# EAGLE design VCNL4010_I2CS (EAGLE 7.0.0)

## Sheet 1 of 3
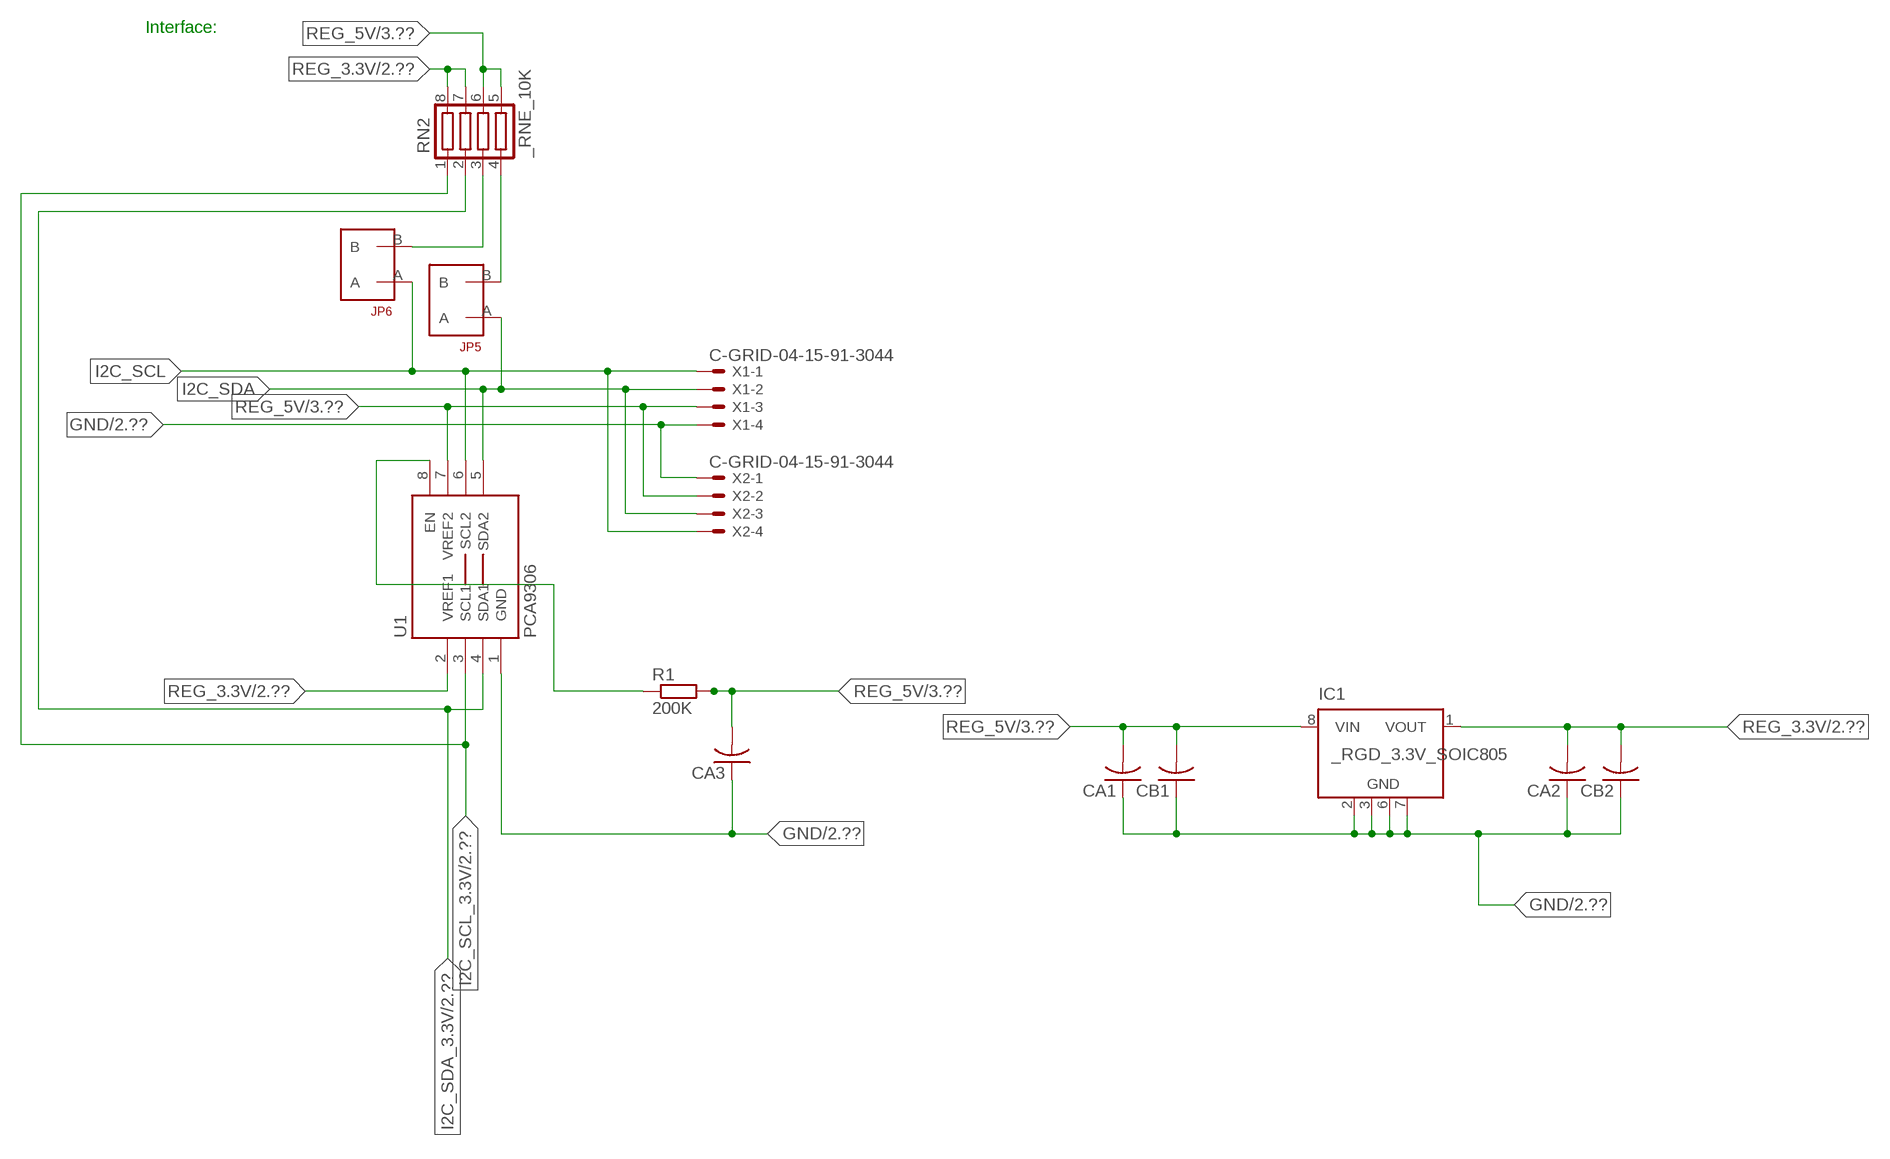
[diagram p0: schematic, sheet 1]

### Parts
CA1  CC1206KRX7R9BB104  [.1UF]
CA2  CC1206KRX7R9BB104  [.1UF]
CA3  CC1206KRX7R9BB104  [.1UF]
CB1  TMK316F106ZL-TC1206K  [TMK316F106ZL-T]
CB2  TMK316F106ZL-TC1206K  [TMK316F106ZL-T]
IC1  _RGD_3.3V_SOIC805  [_RGC_3.3V_SOIC8]
JP5  JUMPER_1X2_2MM  [JUMPER_1X2_2MM]
JP6  JUMPER_1X2_2MM  [JUMPER_1X2_2MM]
R1  200K  RESISTOR_SMT-0603  [R603]
RN2  _RNE_10K  [RNE]
U1  PCA9306  PCA9306_NCD  [PSOP-8]
X1  C-GRID-04-15-91-3044  [15-91-04]
X2  C-GRID-04-15-91-3044  [15-91-04]

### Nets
GND: CA1.1 CA2.1 CA3.1 CB1.1 CB2.1 IC1.2(GND) IC1.3(GND) IC1.6(GND) IC1.7(GND) U1.1(GND) X1.4 X2.1 ; also sheet 2,3
I2C_SCL: JP6.A U1.6(SCL2) X1.1 X2.4
I2C_SCL_3.3V: RN2.1 U1.3(SCL1) ; also sheet 2
I2C_SDA: JP5.A U1.5(SDA2) X1.2 X2.3
I2C_SDA_3.3V: RN2.2 U1.4(SDA1) ; also sheet 2
N$1: JP6.B RN2.3
N$2: JP5.B RN2.4
N$3: R1.1 U1.8(EN)
REG_3.3V: CA2.2 CB2.2 IC1.1(VOUT) RN2.7 RN2.8 U1.2(VREF1) ; also sheet 2
REG_5V: CA1.2 CA3.2 CB1.2 IC1.8(VIN) R1.2 RN2.5 RN2.6 U1.7(VREF2) X1.3 X2.2 ; also sheet 3
Unconnected: IC1.4(NC) IC1.5(NC)

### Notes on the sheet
- Interface:

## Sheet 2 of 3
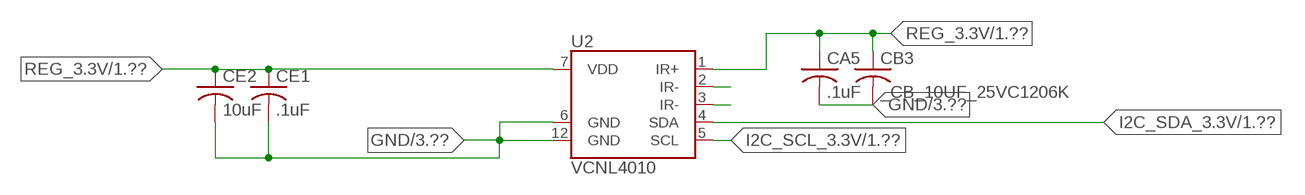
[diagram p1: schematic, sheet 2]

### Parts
CA5  .1uF  CC1206KRX7R9BB104C1206K  [CC1206KRX7R9BB104]
CB3  _CB_10UF_25VC1206K  [_CB_10UF_25V]
CE1  .1uF  _CD_10NF_50VC1206K  [_CD_10NF_50V]
CE2  10uF  CC0603JRNPO8BN1020603  [CC0603JRNPO8BN102]
U2  VCNL4010  VCNL4000  [VCNL4000]

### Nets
GND: CA5.2 CB3.2 CE1.2 CE2.2 U2.6(GND) U2.12(GND) ; also sheet 1,3
I2C_SCL_3.3V: U2.5(SCL) ; also sheet 1
I2C_SDA_3.3V: U2.4(SDA) ; also sheet 1
IR2-: U2.2(IR-)
IR3-: U2.3(IR-)
REG_3.3V: CA5.1 CB3.1 CE1.1 CE2.1 U2.1(IR+) U2.7(VDD) ; also sheet 1

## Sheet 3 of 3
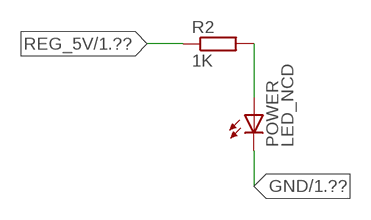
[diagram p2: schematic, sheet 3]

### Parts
POWER  LED_NCD  [CHIPLED_0603]
R2  1K  RESISTOR_SMT-0402  [R402]

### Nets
GND: POWER.C ; also sheet 1,2
N$4: POWER.A R2.2
REG_5V: R2.1 ; also sheet 1

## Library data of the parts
CA1-CA3 CA5 = NCD_ULTIMATE_LIBRARY:CC1206KRX7R9BB104: Capacitor CA .1uF 50V SMT C1206K CC1206KRX7R9BB104
CB1 CB2 = NCD_ULTIMATE_LIBRARY:TMK316F106ZL-T: Capacitor CB 10uF SMT 1206 TMK316F106ZL-T
CB3 = NCD_ULTIMATE_LIBRARY:_CB_10UF_25V: Capacitor 10uF SMT
CE1 = NCD_ULTIMATE_LIBRARY:_CD_10NF_50V: Capacitor 10nF SMT
CE2 = NCD_ULTIMATE_LIBRARY:CC0603JRNPO8BN102: Capacitor CE 1uF SMT CC0603JRNPO8BN102 0603
IC1 = NCD_ULTIMATE_LIBRARY:_RGD_3.3V_SOIC8: Regulator Linear 3.3V Chip Positive VOLTAGE REGULATOR Digikey 497-1199-2-ND/L78L33ACD13TR
JP5 JP6 = NCD_ULTIMATE_CONNECTORS:JUMPER_1X2_2MM
POWER = NCD_ULTIMATE_LIBRARY:LED_NCD: LED Digikey 754-1132-2-ND/APT2012SRCPRV
R1 R2 = NCD_ULTIMATE_LIBRARY:RESISTOR_SMT: NCD Resistor
RN2 = NCD_ULTIMATE_LIBRARY:_RNE_10K: Resistor Array RNE SMT 10K x 4 Single Resistor Source: http://www.ctscorp.com/components/Datasheets/CTSChipArrayDs.pdf Digikey 742C083103JPTR-ND/742C083103JP; OC_FARNELL: unknown; OC_NEWARK: unknown
U1 = NCD_ULTIMATE_LIBRARY:PCA9306_NCD: NCD Bidirectional I2C level shifter. NOT compatible with all available part number pinout schemes- DOUBLE CHECK!!!; PROD_ID: IC-10023
U2 = NCD_ULTIMATE_bhaskar:VCNL4000: Digikey 751-1505-1-ND/VCNL4000-GS08 Fully integrated proximity and ambient light sensor with infrared emitter and I2C interface
X1 X2 = NCD_ULTIMATE_CONNECTORS:C-GRID-04: CONNECTOR 4-Pos I2C wire to board 2.54 mm (0.100") pitch header Digikey WM1342-ND/0015912045; OC_FARNELL: unknown; OC_NEWARK: unknown

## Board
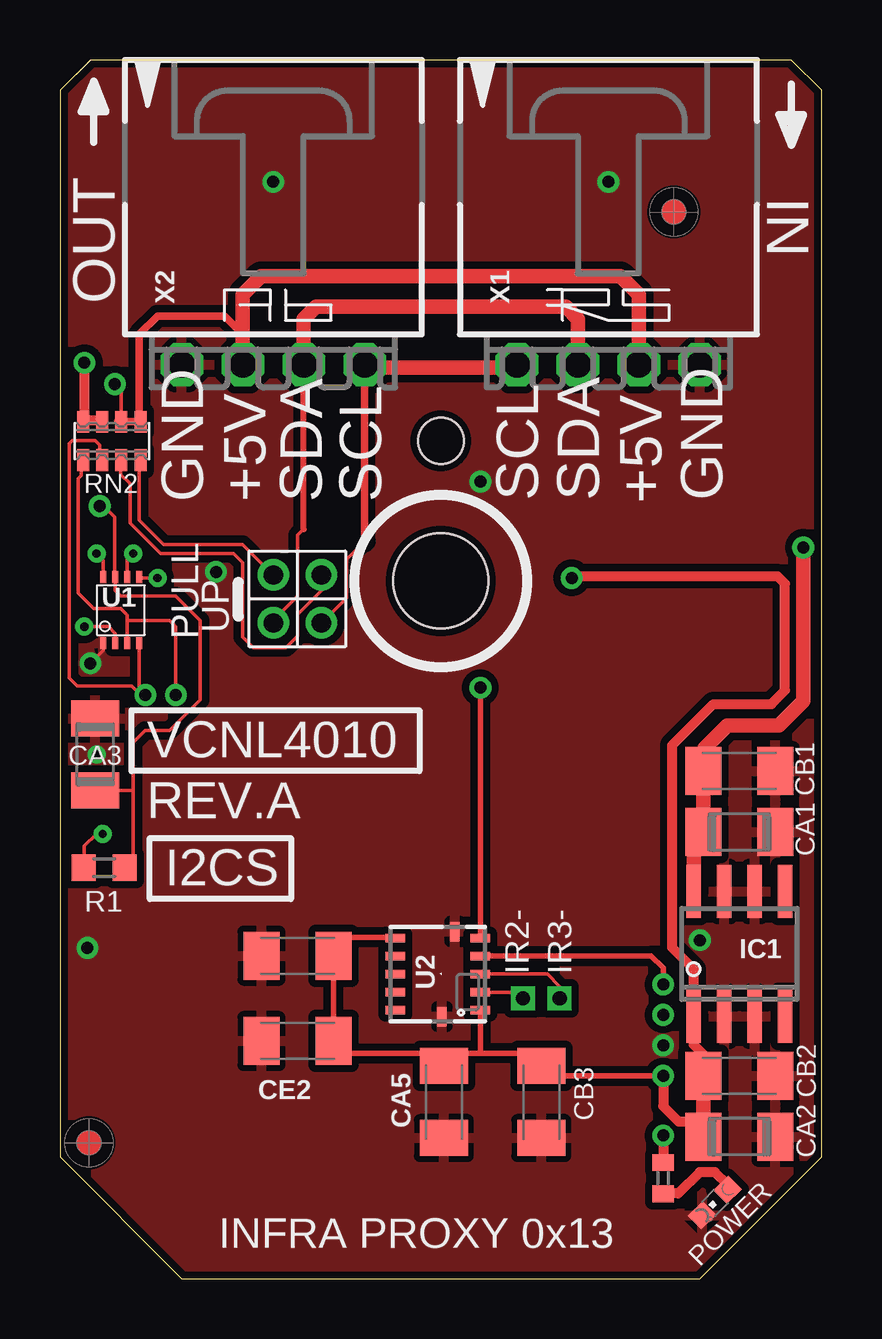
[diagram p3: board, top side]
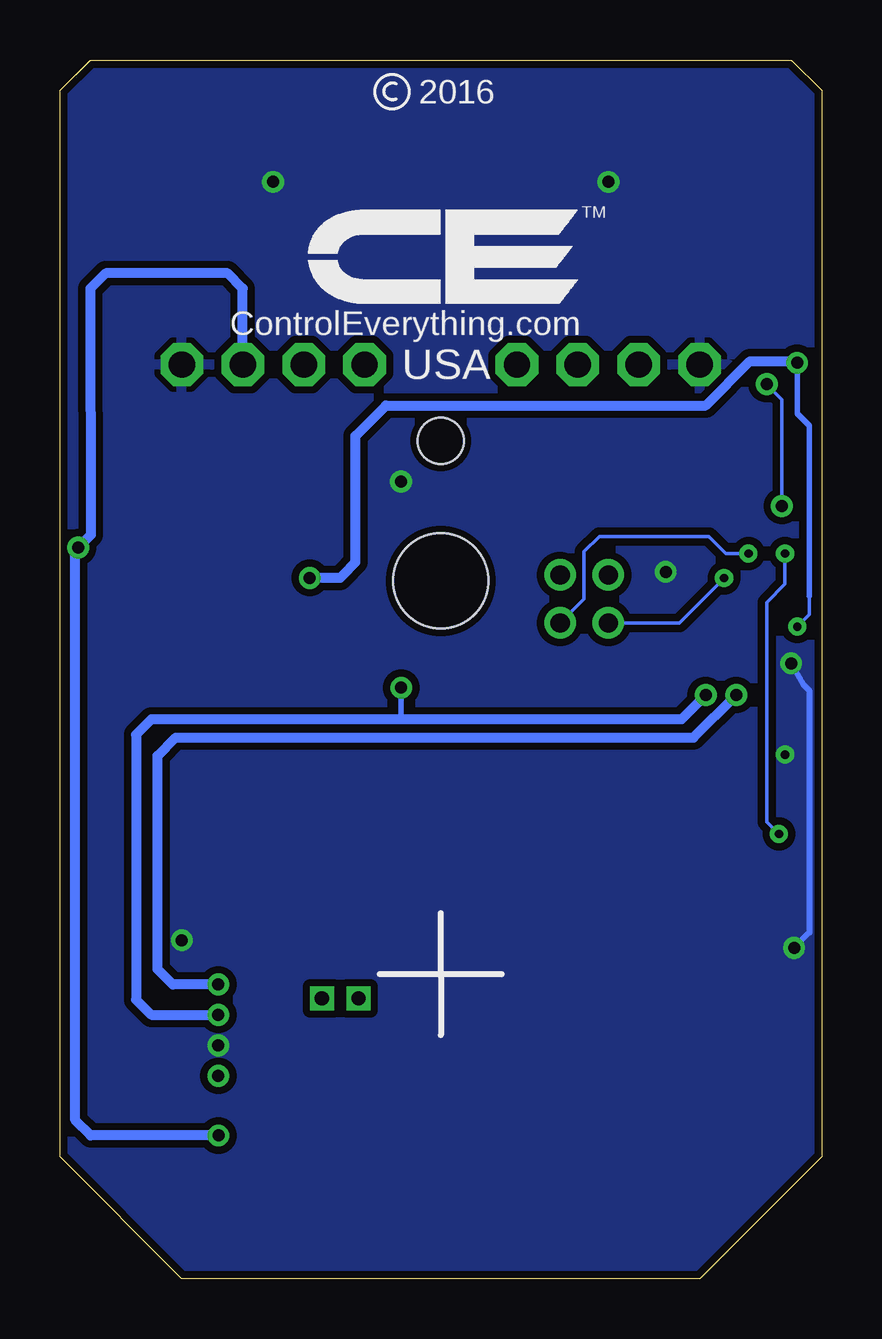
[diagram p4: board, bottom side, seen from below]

Size 31.75 x 50.8 mm. Coordinates in mm from the lower left corner, seen from the top.
Outline: 48 segments
Copper layers (1*16): Top 0.035mm / dielectric 1.5mm / Bottom 0.035mm
Design rules "default": minimum track width 5mil, minimum drill 24mil, track to track 5mil, track to pad 5mil, pad to pad 5mil, via to via 5mil, smd to smd 5mil, copper to edge 10mil, drill to drill 8mil, minimum pad ring 10mil, minimum via ring 8mil, stop-mask expansion 2mil, vias tented up to drill 0mil, thermal gap 10mil
Holes 3.96 mm at 15.88,29.08
Holes 1.91 mm at 15.88,34.93

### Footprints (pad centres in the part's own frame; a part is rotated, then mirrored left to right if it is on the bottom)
.1UF = smd 1.5 x 2: 1 -1.5,0; 2 1.5,0
CC1206KRX7R9BB104 = smd 1.5 x 2: 1 -1.5,0; 2 1.5,0
TMK316F106ZL-T = smd 1.5 x 2: 1 -1.5,0; 2 1.5,0
_CB_10UF_25V = smd 1.5 x 2: 1 -1.5,0; 2 1.5,0
_CD_10NF_50V = smd 1.5 x 2: 1 -1.5,0; 2 1.5,0
CC0603JRNPO8BN102 = smd 1.5 x 2: 1 -1.5,0; 2 1.5,0
_RGC_3.3V_SOIC8 = smd 0.6 x 2.2: 1 -1.905,-2.6; 2 -0.635,-2.6; 3 0.635,-2.6; 4 1.905,-2.6; 5 1.905,2.6; 6 0.635,2.6; 7 -0.635,2.6; 8 -1.905,2.6
JUMPER_1X2_2MM = drill 0.8: A 0,2; B 0,0
CHIPLED_0603 = smd 0.8 x 0.876: A 0,-0.75; C 0,0.75
R603 = smd 1 x 1.1: 1 -0.85,0; 2 0.85,0
R402 = smd 0.7 x 0.9: 1 -0.65,0; 2 0.65,0
RNE = smd 0.5 x 0.9: 1 -1.2,-0.8; 2 -0.4,-0.8; 3 0.4,-0.8; 4 1.2,-0.8; 5 1.2,0.8; 6 0.4,0.8; 7 -0.4,0.8; 8 -1.2,0.8
PSOP-8 = smd 0.25 x 0.5: 1 -0.73,-1.37; 2 -0.23,-1.37; 3 0.27,-1.37; 4 0.77,-1.37; 5 0.77,1.38; 6 0.27,1.38; 7 -0.23,1.38; 8 -0.73,1.38
VCNL4000 = smd 0.35 x 0.805: 1 -1.5,-1.772; 2 -0.75,-1.772; 3 0,-1.772; 4 0.75,-1.772; 5 1.5,-1.772; 7 1.5,1.772; 8 0.75,1.772; 9 0,1.772; 10 -0.75,1.772; 11 -1.5,1.772 | smd 0.805 x 0.4: 6 1.772,-0.715; 12 -1.772,-0.175
15-91-04 = drill 1.1 pad 1.778 octagon: 1 -3.81,-7.62; 2 -1.27,-7.62; 3 1.27,-7.62; 4 3.81,-7.62

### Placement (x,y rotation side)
CA1  28.32,18.62 180 top
CA2  28.32,5.92 180 top
CA3  1.46,21.86 270 top
CA5  16,7.37 270 top
CB1  28.32,21.16 180 top
CB2  28.32,8.46 180 top
CB3  20.07,7.37 270 top
CE1  9.91,13.46 180 top
CE2  9.91,9.91 180 top
IC1  28.32,13.54 0 top
JP5  8.89,29.34 180 top
JP6  10.9,29.34 180 top
POWER  27.3,3.18 135 top
R1  1.84,17.13 0 top
R2  25.15,4.19 270 top
RN2  2.16,34.93 0 top
U1  2.54,27.86 0 top
U2  15.75,12.7 90 top
U$5  [VISION_REF10]  1.21,5.66 90 top
U$28  [VISION_REF10]  25.59,44.46 90 top
X1  22.86,45.72 0 top
X2  8.89,45.72 0 top

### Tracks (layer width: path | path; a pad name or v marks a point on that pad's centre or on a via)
GND  (via drill 0.35, 0.5)
  Top 0.152: CA3.1 1.52,23.42 1.52,23.62 | v1.27,25.65 1.81,26.19 U1.1
  Bottom 0.254: v1.27,25.65 0.76,24.77 0.51,24.51 0.51,14.43 v1.15,13.79
  other vias: 8.89,45.72 22.86,45.72 25.15,9.73 17.53,33.22 26.67,14.11 6.5,29.46 1.52,21.84
  pour Bottom (isolate 0.305): -0.64,5.08 -0.64,49.53 1.27,51.44 30.48,51.44 32.38,49.53 32.38,5.08 26.67,-0.63 5.08,-0.63
  pour Top (isolate 0.305): 4.45,-1.27 -1.27,4.45 -1.27,50.17 0.64,52.07 31.11,52.07 33.02,50.17 33.02,4.45 27.3,-1.27
I2C_SCL  (via drill 0.35)
  Top 0.152: 12.7,30.73 11.94,29.97 11.94,28.38 JP6.A | v3.05,30.23 2.81,29.99 U1.6
  Top 0.305: 12.7,30.73 X2.4
  Top 0.406: X2.4 12.7,37.97 | 19.05,37.97 X1.1
  Top 0.61: 12.7,37.97 19.05,37.97
  Bottom 0.152: JP6.A 9.91,28.33 9.91,30.3 9.27,30.94 4.7,30.94 3.99,30.23 v3.05,30.23
I2C_SCL_3.3V  (via drill 0.5)
  Top 0.152: RN2.1 0.89,34.07 0.89,33.48 0.77,33.35 0.77,28.59 1.41,27.94 2.54,27.94 2.81,27.67 2.81,27.43 | 2.81,27.43 U1.3 | v4.83,24.33 v4.83,24.34 4.83,27.18 4.57,27.43 2.81,27.43
  Top 0.229: U2.5 v17.53,24.64
  Bottom 0.229: v17.53,24.64 17.53,23.32
  Bottom 0.406: v4.83,24.33 5.84,23.32 17.53,23.32 27.94,23.32 28.58,22.68 28.58,11.63 27.94,11 v25.15,11
I2C_SDA  (via drill 0.35)
  Top 0.152: JP5.A 8.89,27.44 9.91,28.45 9.91,30.99 10.16,31.24 | U1.5 3.34,29.21 v4.06,29.21
  Top 0.254: 10.16,31.24 10.16,31.25 X2.3
  Top 0.61: X2.3 10.16,40.01 10.67,40.51 21.09,40.51 21.59,40.01 X1.2
  Bottom 0.152: v4.06,29.21 5.94,27.34 JP5.A
I2C_SDA_3.3V  (via drill 0.5)
  Top 0.152: RN2.2 1.65,34.14 1.65,34.75 1.46,34.94 0.51,34.94 0.38,34.81 0.38,26.37 0.38,26.36 0.38,25.04 0.71,24.71 3,24.71 3.38,24.33 v3.56,24.33 3.31,24.58 U1.4
  Top 0.229: U2.4 17.53,13.46 24.64,13.46 25.15,12.95 v25.15,12.27
  Bottom 0.406: v25.15,12.27 27.05,12.27 27.69,12.9 27.69,21.79 26.93,22.56 5.34,22.56 v3.56,24.33
IR2-  (via drill 0.6)
  Top 0.152: U2.2 17.53,11.94 18.8,11.94 19.05,11.68 v19.3,11.68
IR3-  (via drill 0.6)
  Top 0.152: U2.3 20.32,12.7 20.83,12.19 v20.83,11.68
N$1
  Top 0.152: JP6.B 10.92,29.31 10.92,28.7 9.91,27.69 9.91,26.8 9.42,26.31 8.06,26.31 7.62,26.75 7.62,29.84 7.24,30.23 4.19,30.23 2.92,31.5 2.92,33.15 2.54,33.53 2.54,34.1 RN2.3
  Top 0.305: 2.54,34.02 RN2.3
N$2
  Top 0.152: JP5.B 7.62,30.61 4.32,30.61 3.3,31.62 3.3,34.07 RN2.4
  Top 0.305: 3.37,33.88 RN2.4
N$3  (via drill 0.35)
  Top 0.152: R1.1 1.02,17.16 1.02,18.03 1.52,18.54 v1.78,18.54 | v1.52,30.23 1.81,29.94 U1.8
  Bottom 0.152: v1.78,18.54 2.29,19.05 2.29,28.19 1.52,28.96 v1.52,30.23
N$4
  Top 0.406: POWER.A 27.84,3.92 27.3,4.45 26.67,4.45 25.78,3.56 25.16,3.56 R2.2
REG_3.3V  (via drill 0.35, 0.5)
  Top 0.152: v1.02,27.18 2.03,27.18 2.31,26.9 U1.2
  Top 0.229: 16,9.14 15.75,9.4 11.91,9.4 CE2.1 CE1.1 11.41,13.69 11.94,14.22 13.95,14.22 U2.7 | 17.53,9.4 19.53,9.4 CB3.1 20.47,8.46 v25.15,8.46 | 17.53,9.4 16.26,9.4 16,9.14 | 16,9.14 CA5.1 | U2.1 17.53,9.4
  Top 0.406: CB2.2 26.82,9.35 26.42,9.75 26.42,10.36 | v25.15,8.46 25.15,7.19 25.78,6.55 26.82,6.55 | IC1.1 26.42,12.9 25.53,13.79 25.53,22.24 27.24,23.95 29.66,23.95 30.23,24.52 30.23,28.97 29.91,29.29 21.41,29.29 v21.34,29.21 | 26.52,5.62 CA2.2 | v1.02,38.18 1.02,35.78 | 1.02,35.78 RN2.8 | 1.02,35.78 1.71,35.78 RN2.7
  Top 0.61: CB2.2 26.82,6.55 CA2.2 | 26.42,10.36 IC1.1
  Bottom 0.152: 0.51,28.45 0.51,27.69 v1.02,27.18
  Bottom 0.229: 0.51,28.45 0.51,35.56 1.02,36.07 v1.02,38.18
  Bottom 0.406: v1.02,38.18 1.08,38.24 2.99,38.24 4.83,36.4 18.16,36.4 19.43,35.13 19.43,29.87 19.94,29.34 20.07,29.21 v21.34,29.21
REG_5V  (via drill 0.5)
  Top 0.152: RN2.6 2.56,37.01 v2.29,37.29 | R1.2 3.05,17.49 3.05,20.36 | 3.05,20.36 3.05,22.35 3.56,22.86 4.57,22.86 5.84,24.13 5.84,27.43 4.83,28.45 2.54,28.45 2.31,28.68 U1.7 2.29,29.27 2.29,31.75 1.83,32.21 v1.65,32.21 | CA3.2 3.05,20.36
  Top 0.305: 7.62,39.37 7.5,39.37 | 2.42,35.74 RN2.6 RN2.5 3.31,35.8 3.31,39.37 4.07,40.13 6.86,40.13 7.62,39.37 | X2.2 7.62,39.37
  Top 0.406: v25.15,5.97 R2.1
  Top 0.61: X2.2 7.62,41.02 8.38,41.78 23.37,41.78 24.13,41.02 X1.3 | IC1.8 26.42,18.21 CA1.2 CB1.2 26.86,21.2 26.86,22.11 27.82,23.06 29.98,23.06 30.99,24.08 v30.99,30.48
  Bottom 0.152: v1.65,32.21 1.65,36.65 v2.29,37.29
  Bottom 0.406: X1.3 24.13,41.28 24.77,41.91 29.84,41.91 30.48,41.27 30.47,31 v30.99,30.48 31.11,30.36 31.11,6.6 30.48,5.97 v25.15,5.97

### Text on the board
tNames: IN | OUT | GND | +5V | SDA | SCL | SCL | SDA | +5V | GND | PULL | UP | VCNL4010 | REV.A | I2CS | IR2- | IR3- | INFRA PROXY 0x13
bNames: 2016 | TM | ControlEverything.com | USA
